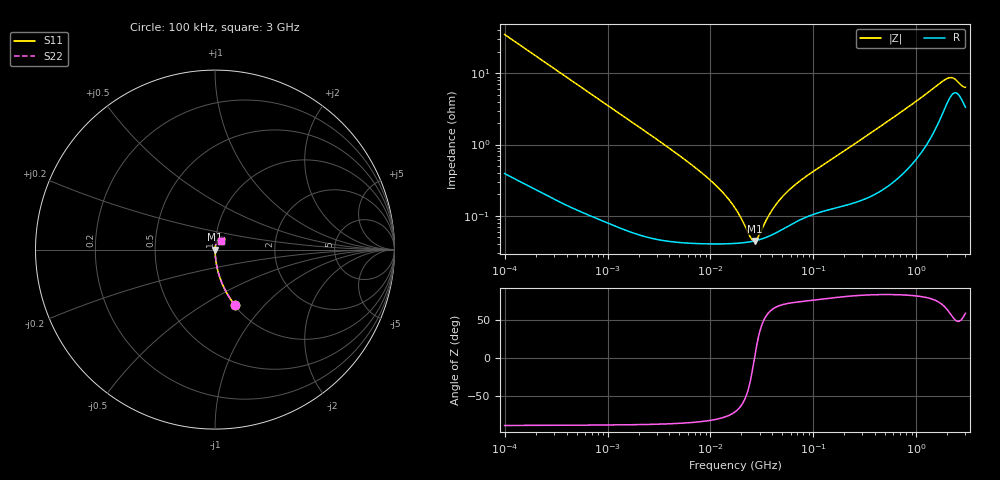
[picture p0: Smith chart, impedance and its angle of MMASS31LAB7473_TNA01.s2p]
! MMASS31LAB7473_TNA01  S-PARAMETER MODEL  ( Standard Model )
! Model Generated by TAIYO YUDEN Corporation (http://www.ty-top.com)
! Version 1.0
! TAIYO YUDEN Control No. 220601
! Copyright(c) 2018 TAIYO YUDEN CO.,LTD. All Rights Reserved.
! Product Description (link to TY-COMPAS)
! https://ds.yuden.co.jp/TYCOMPAS/or/detail?pn=MMASS31LAB7473KTNA01&u=M
! Products Name : Multilayer Ceramic Capacitors
! Characteristics :
!  Capacitance : 0.047 [uF] , Rated Voltage : 630 [V] , TCC : X7R
!  Case Size : 3.2 x 1.6 / 0.126 x 0.063 [mm/inch] , Thickness : 1.6 / 0.063 [mm/inch]
!  (Conditions: Temperature = 25 [degC] , DC Bias Voltage = 0 [V])
! External Node Assignments :
!  1  o---| |---o  2
! GND o---------o GND
! Frequency Range : 100kHz  -  3GHz  [ 401 STEP ]
# MHZ S RI R 50
! Freq[MHz].  S11 Real  S11 Imag  S21 Real  S21 Imag  S12 Real  S12 Imag  S22 Real  S22 Imag
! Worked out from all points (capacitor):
!   401 points, 100 kHz to 3 GHz, reference 50 ohm
!   read as one part in series: C = 45.2 nF near 105.3 kHz
!   lowest |Z| = 44.4 mohm at 26.84 MHz (marker M1)
!   series resonance near 26.84 MHz, so ESL is about 780 pH
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0.1  0.1127 -0.3107  0.8873 0.3107  0.8873 0.3107  0.1127 -0.3107
0.228123  0.0254 -0.1507  0.9746 0.1507  0.9746 0.1507  0.0254 -0.1507
0.562235  0.0051 -0.0629  0.9949 0.0629  0.9949 0.0629  0.0051 -0.0629
3.161081  0.000586 -0.0112  0.9994 0.0112  0.9994 0.0112  0.000586 -0.0112
6.178009  0.000442 -0.00554  0.9996 0.00554  0.9996 0.00554  0.000442 -0.00554
9.824692  0.000413 -0.00319  0.9996 0.00319  0.9996 0.00319  0.000413 -0.00319
13.7349  0.000407 -0.00195  0.9996 0.00195  0.9996 0.00195  0.000407 -0.00195
17.7727  0.000411 -0.00115  0.9996 0.00115  0.9996 0.00115  0.000411 -0.00115
24.21403  0.000431 -0.000279  0.9996 0.000279  0.9996 0.000279  0.000431 -0.000279
25.49486  0.000437 -0.000139  0.9996 0.000139  0.9996 0.000139  0.000437 -0.000139
26.84345  0.000443 7.27e-07  0.9996 -7.27e-07  0.9996 -7.27e-07  0.000443 7.27e-07
29.00125  0.000456 0.00021  0.9995 -0.00021  0.9995 -0.00021  0.000456 0.00021
37.52708  0.000521 0.000914  0.9995 -0.000914  0.9995 -0.000914  0.000521 0.000914
47.32384  0.000617 0.00157  0.9994 -0.00157  0.9994 -0.00157  0.000617 0.00157
64.47533  0.000794 0.0025  0.9992 -0.0025  0.9992 -0.0025  0.000794 0.0025
97.38194  0.00105 0.00396  0.999 -0.00396  0.999 -0.00396  0.00105 0.00396
547.5153  0.00315 0.0217  0.9969 -0.0217  0.9969 -0.0217  0.00315 0.0217
1281.618  0.0128 0.0509  0.9872 -0.0509  0.9872 -0.0509  0.0128 0.0509
1935.725  0.0386 0.0699  0.9614 -0.0699  0.9614 -0.0699  0.0386 0.0699
2259.438  0.053 0.0624  0.947 -0.0624  0.947 -0.0624  0.053 0.0624
2776.789  0.0428 0.0477  0.9572 -0.0477  0.9572 -0.0477  0.0428 0.0477
3000  0.035 0.0506  0.965 -0.0506  0.965 -0.0506  0.035 0.0506
